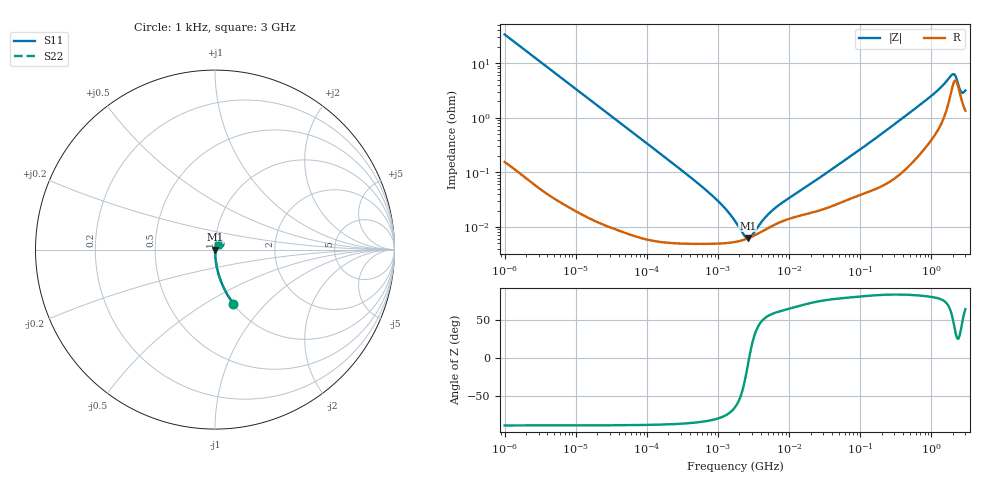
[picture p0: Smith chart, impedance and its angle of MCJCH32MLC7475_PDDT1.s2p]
! MCJCH32MLC7475_PDDT1  S-PARAMETER MODEL  ( Standard Model )
! Model Generated by TAIYO YUDEN Corporation (http://www.ty-top.com)
! Version 1.0
! TAIYO YUDEN Control No. 220601
! Copyright(c) 2016 TAIYO YUDEN CO.,LTD. All Rights Reserved.
! Product Description (link to TY-COMPAS)
! https://ds.yuden.co.jp/TYCOMPAS/or/detail?pn=MCJCH32MLC7475KPDDT1&u=M
! Products Name : Multilayer Ceramic Capacitors
! Characteristics :
!  Capacitance : 4.7 [uF] , Rated Voltage : 100 [V] , TCC : X7S
!  Case Size : 3.2 x 2.5 / 0.126 x 0.098 [mm/inch] , Thickness : 2.5 / 0.098 [mm/inch]
!  (Conditions: Temperature = 25 [degC] , DC Bias Voltage = 0 [V])
! External Node Assignments :
!  1  o---| |---o  2
! GND o---------o GND
! Frequency Range : 1kHz  -  3GHz  [ 401 STEP ]
# MHZ S RI R 50
! Freq[MHz].  S11 Real  S11 Imag  S21 Real  S21 Imag  S12 Real  S12 Imag  S22 Real  S22 Imag
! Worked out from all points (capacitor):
!   401 points, 1 kHz to 3 GHz, reference 50 ohm
!   read as one part in series: C = 4.74 uF near 1.077 kHz
!   lowest |Z| = 6.28 mohm at 2.61 MHz (marker M1)
!   series resonance near 2.742 MHz, so ESL is about 710 pH
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0.001  0.1022 -0.3006  0.8978 0.3006  0.8978 0.3006  0.1022 -0.3006
0.001685  0.039 -0.1913  0.961 0.1913  0.961 0.1913  0.039 -0.1913
0.00306  0.0124 -0.1085  0.9876 0.1085  0.9876 0.1085  0.0124 -0.1085
0.01216  0.000939 -0.0277  0.9991 0.0277  0.9991 0.0277  0.000939 -0.0277
0.147855  5.88e-05 -0.00229  0.9999 0.00229  0.9999 0.00229  5.88e-05 -0.00229
0.791611  4.93e-05 -0.000394  1 0.000394  1 0.000394  4.93e-05 -0.000394
1.238299  5.05e-05 -0.000218  0.9999 0.000218  0.9999 0.000218  5.05e-05 -0.000218
1.732051  5.32e-05 -0.000117  0.9999 0.000117  0.9999 0.000117  5.32e-05 -0.000117
2.010629  5.54e-05 -7.72e-05  0.9999 7.72e-05  0.9999 7.72e-05  5.54e-05 -7.72e-05
2.610246  6.16e-05 -1.18e-05  0.9999 1.18e-05  0.9999 1.18e-05  6.16e-05 -1.18e-05
3.651041  7.57e-05 6.72e-05  0.9999 -6.72e-05  0.9999 -6.72e-05  7.57e-05 6.72e-05
4.919932  9.38e-05 0.000135  0.9999 -0.000135  0.9999 -0.000135  9.38e-05 0.000135
6.629817  0.000114 0.000202  0.9999 -0.000202  0.9999 -0.000202  0.000114 0.000202
21.06097  0.000184 0.000617  0.9998 -0.000617  0.9998 -0.000617  0.000184 0.000617
256.0921  0.000708 0.00644  0.9993 -0.00644  0.9993 -0.00644  0.000708 0.00644
1056.143  0.00501 0.0262  0.995 -0.0262  0.995 -0.0262  0.00501 0.0262
1917.819  0.0331 0.0484  0.9669 -0.0484  0.9669 -0.0484  0.0331 0.0484
2066.299  0.0446 0.0407  0.9554 -0.0407  0.9554 -0.0407  0.0446 0.0407
2144.796  0.0472 0.0328  0.9528 -0.0328  0.9528 -0.0328  0.0472 0.0328
2584.342  0.0239 0.0172  0.9761 -0.0172  0.9761 -0.0172  0.0239 0.0172
2784.426  0.0175 0.0222  0.9825 -0.0222  0.9825 -0.0222  0.0175 0.0222
3000  0.0141 0.0278  0.9859 -0.0278  0.9859 -0.0278  0.0141 0.0278
